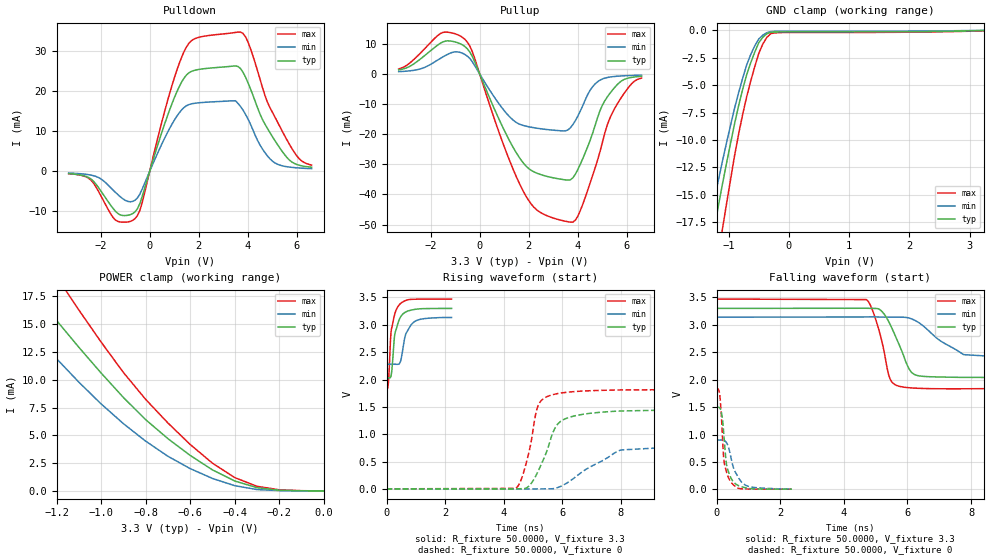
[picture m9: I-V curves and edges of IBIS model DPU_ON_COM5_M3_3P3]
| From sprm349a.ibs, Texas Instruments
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|   Model Cell DPU_ON_COM5_M3_3P3
|DPU_ON_COM5_M3_3P3
[Model]   DPU_ON_COM5_M3_3P3
Model_type   I/O
Polarity   Non-Inverting
Enable   Active-Low
Vinl =  0.8V
Vinh =  2V
Cref =  15.0000pF
Rref =  100.0000M
Vref =  0V
Vmeas =  1.65
C_comp   1.482056p   1.446471p   1.52328p
[Model Spec]
Vinl   0.8V   0.8V   0.8V
Vinh   2V   2V   2V
[Temperature Range]   25   105   0
[Voltage Range]   3.3   3.14   3.47
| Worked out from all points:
|   slope of the pulldown table from 0 to 0.495 V, typ, clamps not added: 50.8 ohm
|   slope of the pullup table from 0 to 0.495 V, typ, clamps not added: 51.2 ohm
|   GND clamp passes 1 mA (typ) near -0.48 V on its own axis
|   POWER clamp passes 1 mA (typ) near -0.41 V on its own axis
|   rising waveform, R_fixture 50.0000, V_fixture 3.3: 20-80 % time 200ps typ, 272ps min, 167ps max; typ from 2.03 V to 3.3 V
|   rising waveform, R_fixture 50.0000, V_fixture 0: 20-80 % time 702ps typ, 1.64ns min, 425ps max; typ from 0.003 V to 1.49 V
|   falling waveform, R_fixture 50.0000, V_fixture 3.3: 20-80 % time 555ps typ, 1.49ns min, 406ps max; typ from 3.3 V to 2.04 V
|   falling waveform, R_fixture 50.0000, V_fixture 0: 20-80 % time 187ps typ, 320ps min, 151ps max; typ from 1.5 V to 0.005 V
[POWER_clamp]
|   voltage   I(typ)   I(min)   I(max)
-3.3V     79.08mA    60.56mA    96.76mA
-1.467V   22.4mA     17.93mA    27.7mA
-1.433V   21.45mA    17.16mA    26.59mA
-1.3V     17.85mA    14.11mA    22.34mA
-1.267V   17.01mA    13.37mA    21.32mA
-1.133V   13.73mA    10.5mA     17.28mA
-900mV    8.413mA    6.059mA    10.66mA
-800mV    6.415mA    4.484mA    8.242mA
-500mV    1.895mA    1.125mA    2.5mA
-400mV    896.1uA    472.4uA    1.202mA
-300mV    292.5uA    123.4uA    418.7uA
0V        123.6nA    125.9nA    560.1nA
[Pulldown]
|   voltage   I(typ)   I(min)   I(max)
-3.3V     -543.5uA   -399.7uA   -549.7uA
-2.4V     -1.844mA   -904.9uA   -2.118mA
-1.4V     -9.906mA   -5.191mA   -12.13mA
-600mV    -10.12mA   -7.213mA   -11.81mA
-300mV    -6.174mA   -4.366mA   -7.707mA
900mV     16.8mA     11.71mA    21.29mA
1.5V      24.11mA    16.42mA    31.12mA
3.6V      26.24mA    17mA       34.84mA
4V        22.29mA    13.21mA    32.47mA
5V        8.731mA    2.592mA    14.83mA
6V        1.731mA    900.9uA    3.861mA
6.6V      1.052mA    699uA      1.588mA
[Pullup]
|   voltage   I(typ)   I(min)   I(max)
-3.3V     1.325mA    743.3uA    1.642mA
-1.6V     10.17mA    5.149mA    13.4mA
-600mV    9.081mA    6.451mA    11.47mA
-300mV    5.824mA    4.052mA    7.406mA
1.1V      -20.32mA   -13.16mA   -26.27mA
1.9V      -30.67mA   -17.37mA   -40.73mA
2.5V      -33.44mA   -18.22mA   -46.1mA
3.7V      -35.15mA   -17.87mA   -49.23mA
4.2V      -28.16mA   -10.56mA   -43.32mA
5.2V      -7.671mA   -1.199mA   -16.95mA
6V        -1.51mA    -579.6uA   -5.193mA
6.6V      -789.4uA   -430.3uA   -1.374mA
[GND_clamp]
|   voltage   I(typ)   I(min)   I(max)
-3.3V     -90.84mA   -70.66mA   -109.9mA
-1.367V   -22.38mA   -18.9mA    -27.63mA
-1.3V     -20.12mA   -17.12mA   -25.11mA
-1.233V   -18mA      -15.36mA   -22.74mA
-1.1V     -13.98mA   -11.9mA    -18.08mA
-1.033V   -12.11mA   -10.25mA   -15.82mA
-900mV    -8.507mA   -7.094mA   -11.42mA
-700mV    -4.047mA   -3.151mA   -6.062mA
-500mV    -1.132mA   -785.8uA   -2.111mA
-366.7mV  -307.9uA   -209.6uA   -647.7uA
-166.7mV  -139.7uA   -74.6uA    -197.5uA
3.233V    -8.644uA   9.327uA    -37.99uA
[Ramp]
| variable   typ   min   max
dV/dt_f  0.7672372/0.5591447n  0.5265868/1.288437n   0.9969463/0.4101334n
dV/dt_r  0.8977249/0.7047203n  0.5375279/1.657537n   1.103651/0.4256236n
R_load = 50
[Rising Waveform]
R_fixture = 50.0000
V_fixture = 3.3
V_fixture_min = 3.14
V_fixture_max = 3.47
|   time   V(typ)   V(min)   V(max)
0s        2.029V     2.278V     1.821V
60ps      2.03V      2.28V      1.92V
135ps     2.039V     2.281V     2.714V
165ps     2.099V     2.28V      2.913V
270ps     2.776V     2.28V      3.174V
420ps     3.076V     2.283V     3.356V
495ps     3.156V     2.368V     3.396V
645ps     3.23V      2.811V     3.442V
900ps     3.274V     3.035V     3.465V
2.22ns    3.298V     3.134V     3.469V
[Rising Waveform]
R_fixture = 50.0000
V_fixture = 0
V_fixture_min = 0
V_fixture_max = 0
|   time   V(typ)   V(min)   V(max)
0s        3.341mV    2.039mV    4.112mV
4.41ns    4.004mV    1.016mV    17.27mV
4.71ns    10.73mV    -377.9uV   363.4mV
5.115ns   262.3mV    3.073mV    1.426V
5.265ns   433mV      3.354mV    1.606V
5.94ns    1.236V     49.19mV    1.753V
7.245ns   1.4V       484.8mV    1.801V
7.995ns   1.426V     714.6mV    1.81V
16.95ns   1.478V     869.7mV    1.826V
115.4ns   1.491V     891.1mV    1.838V
[Falling Waveform]
R_fixture = 50.0000
V_fixture = 3.3
V_fixture_min = 3.14
V_fixture_max = 3.47
|   time   V(typ)   V(min)   V(max)
0s        3.3V       3.14V      3.47V
4.71ns    3.303V     3.143V     3.46V
5.07ns    3.295V     3.143V     2.975V
5.4ns     3.073V     3.14V      2.115V
5.49ns    2.968V     3.14V      1.977V
6.045ns   2.203V     3.126V     1.854V
6.585ns   2.057V     2.937V     1.839V
7.77ns    2.042V     2.457V     1.835V
12.54ns   2.038V     2.288V     1.849V
122.5ns   2.036V     2.275V     1.822V
[Falling Waveform]
R_fixture = 50.0000
V_fixture = 0
V_fixture_min = 0
V_fixture_max = 0
|   time   V(typ)   V(min)   V(max)
0s        1.498V     899.1mV    1.839V
105ps     1.482V     900.7mV    1.707V
180ps     1.311V     900.9mV    1.031V
210ps     1.141V     897.6mV    699.3mV
240ps     925.9mV    891.2mV    497mV
315ps     449.6mV    850.5mV    315mV
450ps     212.3mV    590mV      137.8mV
585ps     107mV      320.5mV    56.55mV
915ps     29.59mV    75.23mV    8.17mV
2.37ns    4.969mV    8.689mV    4.646mV
